{attribute 'no-analysis'}
FUNCTION_BLOCK FB_DirectControl EXTENDS FB_Control
VAR
	_eControlState: E_DirectControlState; (*State of control state machine*)
END_VAR

METHOD Execute : BOOL
VAR
	bTestOk: BOOL; (*Used to cache the return value of the last '_OperativeTest' or '_DynamicTest' method call*)
	eError: E_AcsiServiceError; (*Used to cache the returned error of the last '_OperativeTest' or '_DynamicTest' method call*)
	tValue: T_UtcTime; (*Used to cache the current system time for 'tOpOk'*)
END_VAR
IF (_ipCtrl <> 0) AND_THEN (_ipCtrl.ipOper <> 0) THEN
	(* Initialize function block in the first cycle *)
	IF NOT bInit THEN
		_Init();
		bInit:=TRUE;
	END_IF

	CASE _eControlState OF
		E_DirectControlState.Ready:
			(* Check if ControlState changed in the last cycle *)
			IF bNewState THEN
				bNewState:=FALSE;
				_Reset();
			END_IF
			(* Check if a valid Oper_req was received *)
			IF bOperReq THEN
				bOperReq:=FALSE;
				(* Go to next ControlState *)
				_eControlState:=E_DirectControlState.PerformTest;
				bNewState:=TRUE;
			END_IF

		E_DirectControlState.PerformTest:
			(* Check if ControlState changed in the last cycle *)
			IF bNewState THEN
				bNewState:=FALSE;
				(* Set 'opRcvd' *)
				IF (_ipCtrl.ipOpRcvd <> 0) THEN
					_ipCtrl.ipOpRcvd.bValue:=TRUE;
				END_IF
			END_IF
			(* Trigger the operative test until it is finished *)
			IF _OperativeTest(bOperativeTestOk=>bTestOk, eError=>eError) THEN
				(* Reset 'opRcvd' *)
				IF (_ipCtrl.ipOpRcvd <> 0) THEN
					_ipCtrl.ipOpRcvd.bValue:=FALSE;
				END_IF
				IF bTestOk THEN
					(* Go to next ControlState *)
					_eControlState:=E_DirectControlState.WaitForExecution;
				ELSE
					fbCompletion.SetCompleted();
					fbCompletion.eServiceError:=eError;
					(* Go back to ControlState 'Ready' *)
					_eControlState:=E_DirectControlState.Ready;
				END_IF
				bNewState:=TRUE;
			END_IF

		E_DirectControlState.WaitForExecution:
			(* Check if ControlState changed in the last cycle *)
			IF bNewState THEN
				bNewState:=FALSE;
			END_IF
			(* Trigger the dynamic test until it is finished *)
			IF _DynamicTest(bDynamicTestOk=>bTestOk, eError=>eError) THEN
				fbCompletion.SetCompleted();
				IF bTestOk THEN
					(* Go to next ControlState *)
					IF (_ipBehVal <> 0) AND_THEN ((_ipBehVal.eValue = E_AcsiBeh.TestBlocked) OR_ELSE (_ipBehVal.eValue = E_AcsiBeh.OnBlocked)) THEN
						_eControlState:=E_DirectControlState.MirrorBlockedCommand;
					ELSE
						_eControlState:=E_DirectControlState.Operate;
					END_IF
				ELSE
					fbCompletion.eServiceError:=eError;
					(* Go back to ControlState 'Ready' *)
					_eControlState:=E_DirectControlState.Ready;
				END_IF
				bNewState:=TRUE;
			END_IF

		E_DirectControlState.Operate:
			(* Check if ControlState changed in the last cycle *)
			IF bNewState THEN
				bNewState:=FALSE;
				(* Set 'opOk' *)
				IF (_ipCtrl.ipOpOk <> 0) THEN
					_ipCtrl.ipOpOk.bValue:=TRUE;
				END_IF
				(* Set 'tOpOk' *)
				IF (_ipCtrl.ipTOpOk <> 0) AND_THEN (_ipCurrentAA <> 0) AND_THEN (_ipCurrentAA.GetSystemTime(tT=>tValue)) THEN
					_ipCtrl.ipTOpOk.tValue:=tValue;
				END_IF
			END_IF
			(* Update value *)
			_SetValue(uCtlVal:=_ipCtrl.ipOper.uCtlVal, ipCtlVal_AV:=_ipCtrl.ipOper.ipCtlVal_AnalogueValue);
			(* Update Timestamp 't' *)
			_UpdateTimestampValue(ipAA:=_ipCurrentAA);

			(* Reset 'opOk' *)
			IF (_ipCtrl.ipOpOk <> 0) THEN
				_ipCtrl.ipOpOk.bValue:=FALSE;
			END_IF
			(* Go back to ControlState 'Ready' *)
			_eControlState:=E_DirectControlState.Ready;
			bNewState:=TRUE;

		E_DirectControlState.MirrorBlockedCommand:
			(* Check if ControlState changed in the last cycle *)
			IF bNewState THEN
				bNewState:=FALSE;
				(* Set 'opOk' *)
				IF (_ipCtrl.ipOpOk <> 0) THEN
					_ipCtrl.ipOpOk.bValue:=TRUE;
				END_IF
				(* Set 'tOpOk' *)
				IF (_ipCtrl.ipTOpOk <> 0) AND_THEN (_ipCurrentAA <> 0) AND_THEN (_ipCurrentAA.GetSystemTime(tT=>tValue)) THEN
					_ipCtrl.ipTOpOk.tValue:=tValue;
				END_IF
			END_IF
			(* Reset 'opOk' *)
			IF (_ipCtrl.ipOpOk <> 0) THEN
				_ipCtrl.ipOpOk.bValue:=FALSE;
			END_IF
			(* Go back to ControlState 'Ready' *)
			_eControlState:=E_DirectControlState.Ready;
			bNewState:=TRUE;
	END_CASE
END_IF

(* Monitor transmission of LastApplError *)
CASE _nLastApplErrorReqState OF
	0:	RETURN;
	1:
		IF (_ipLastApplErrorReq <> 0) THEN
			Execute:=_ipLastApplErrorReq.Execute();
			IF NOT _ipLastApplErrorReq.IsBusy() THEN
				IF _ipLastApplErrorReq.IsCompleted() THEN
					SUPER^.SetCompleted();
				ELSE
					SUPER^.CopyFrom(ipSource:=_ipLastApplErrorReq);
				END_IF
				_nLastApplErrorReqState:=0;
			END_IF
		END_IF
END_CASE
END_METHOD

METHOD OnCompletionWaitEvent : BOOL
VAR_INPUT
	ipDai: I_AcsiDataAccessInfoClass;
	ipData: I_AcsiCommonDataClass;
	eFc: E_AcsiFc;
END_VAR
VAR_OUTPUT
	ipResult: I_AcsiServiceResultClass := fbCompletion;
END_VAR
VAR
	eServiceError: E_AcsiServiceError;
END_VAR
fbCompletion.SetCompleted();
IF (ipDai = 0) OR_ELSE (ipData = 0) THEN
	fbCompletion.eServiceError:=E_AcsiServiceError.AccessViolation;
	RETURN;
END_IF

(* Check if an Operate request is received *)
IF (ipDai.eService = E_AcsiServiceType.SetDataValues) AND_THEN (ipData.sObjectName = 'Oper') THEN
	ScsmAssociation_From_Dai(in:=ipDai, out=>_ipCurrentAA);
	fbCompletion.SetBusy();
	bOperReq:=TRUE;
	OnCompletionWaitEvent:=TRUE;
END_IF
END_METHOD

(*Implementation of user application data update event method.*)
METHOD OnSetVPreEvent : E_AcsiServiceError
VAR_INPUT
	ipDai: I_AcsiDataAccessInfoClass; (*Additional data access info*)
	ipMemory: I_AnyMemoryBuffer; (*Interface pointer to buffer containig new value data*)
	ipData: I_AcsiCommonDataClass; (*Interface pointer to data object*)
	eFc: E_AcsiFc; (*Functional constraint*)
END_VAR
VAR_OUTPUT
	ipLastApplError: I_AcsiDATypeLastApplError; (*IF <> 0 => send LastApplError request*)
END_VAR
VAR
	ipAA: I_ScsmAssociationClass; (*Interface pointer to application association*)
END_VAR
IF (eFc = E_AcsiFc.CO) AND_THEN (_ipCtrl <> 0) AND_THEN (ipDai <> 0) AND_THEN (ipDai.Write) AND_THEN (ipDai.ipAccessData <> 0) AND_THEN ScsmAssociation_From_Dai(in:=ipDai, out=>ipAA) THEN
	IF (_ipCtrl.ipOper <> 0) AND_THEN (_ipCtrl.ipOper.ipOrigin <> 0) AND_THEN (_ipCtrl.ipOper.ipCtlNum <> 0) THEN
		(* Check for invalid write attemps to prevent 'Oper' from being overwritten while a control request is being executed *)
		IF (ipDai.ipAccessData.sObjectName = 'Oper') THEN
			(* Only allow 'Oper' requests in state 'Ready' *)
			IF (_eControlState <> E_DirectControlState.Ready) THEN
				ipLastApplError:=ipAA.SetAdditionalCauseDiag(ipCtrlData:=_ipCtrl.ipOper, eError:=E_AcsiApplError.NoError, stOrigin:=_ipCtrl.ipOper.ipOrigin.stOrigin, nCtlNum:=_ipCtrl.ipOper.ipCtlNum.nValue, eAddCause:=E_AcsiApplAddCause.CommandAlreadyInExecution);
				OnSetVPreEvent:=E_AcsiServiceError.AccessViolation;
			END_IF
		ELSE
			(* Don't allow write access to subdata of 'Oper' *)
			ipLastApplError:=ipAA.SetAdditionalCauseDiag(ipCtrlData:=_ipCtrl.ipOper, eError:=E_AcsiApplError.NoError, stOrigin:=_ipCtrl.ipOper.ipOrigin.stOrigin, nCtlNum:=_ipCtrl.ipOper.ipCtlNum.nValue, eAddCause:=E_AcsiApplAddCause.NotSupported);
			OnSetVPreEvent:=E_AcsiServiceError.AccessViolation;
		END_IF
	END_IF
END_IF
END_METHOD

END_FUNCTION_BLOCK
